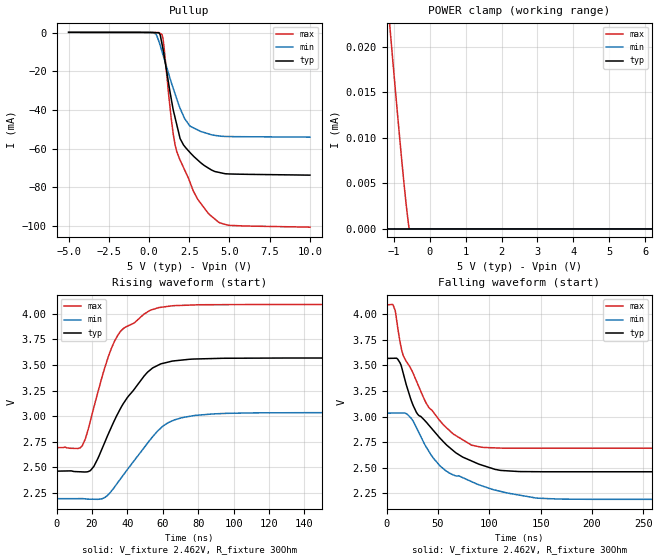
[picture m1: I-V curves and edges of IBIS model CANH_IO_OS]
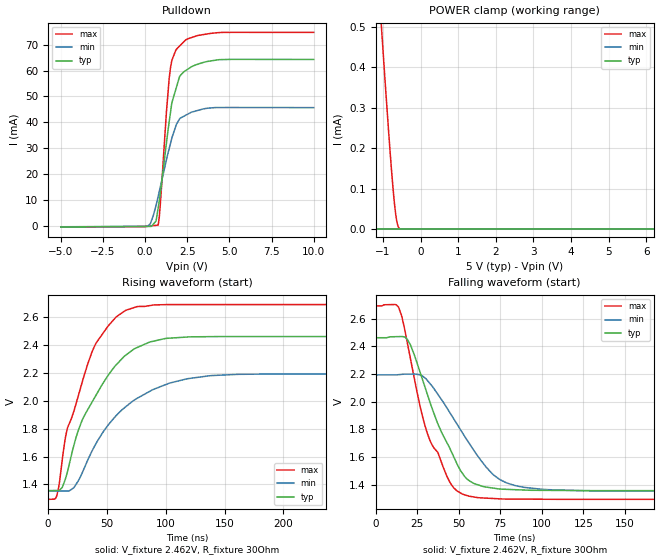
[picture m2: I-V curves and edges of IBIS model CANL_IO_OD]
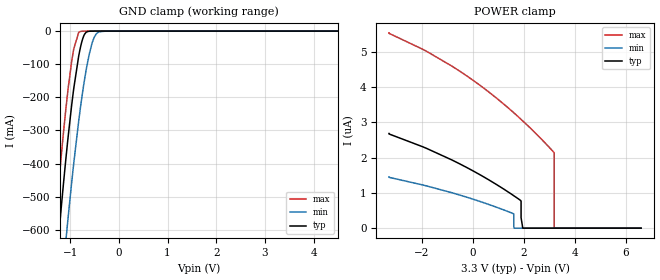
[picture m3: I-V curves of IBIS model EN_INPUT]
| Texas Instruments Incorporated
| TCAN1043Ax-Q1 Fault Protected CAN Transceiver with CAN FD
| Marketing part#   Digital Voltage Range   Package-type   #pins
| TCAN1043A-Q1   2.8V - 40V   SOIC , VSON   14
[IBIS Ver]   4.1
[File name]   tcan1043a-q1.ibs
[File Rev]   1.0
[Date]   12/13/2021
[Source]
| Texas Instruments Incorporated.
| Analog-eLab Design Center, HPA
| 12500 TI Blvd
| Dallas, TX -75243
[Notes]   Revision History:
| Rev 1.0: 12/13/2021
| - Initial version of the model
| - Model generated from simulations in SPECTRE
| - Model matched to SPICE simulation
| - C_comp although listed in numerical order of value are
|   obtained from varying PVT conditions. For PVT conditions for
|   each specific value refer the buffer description under
|   respective [Model]. IBIS model user is responsible for using
|   appropriate C_comp to simulate for Signal Integrity.
| - Notes regarding combined Non-monotonicity of various models
|   have been reviewed and considered minor and can be ignored.
| - For IBIS simulation of CANH-CANL differential pair, it is recommended
|   to use a capacitor(C) at common mode terminal with C >= 4.7nF
[Disclaimer]
| This model is designed as an aid for customers of Texas Instruments.
| TI and its licensors and suppliers make no warranties, either expressed
| or implied, with respect to this  model, including the warranties of
| merchantability or fitness for a particular purpose. The model is
| provided solely on an "as is" basis. The entire risk as to its quality
| and performance is with the customer.
[Copyright]
(C) Copyright 2017 Texas Instruments Incorporated.All rights reserved.
|   TCAN1043A-Q1_D
[Component]   TCAN1043A-Q1_D
[Manufacturer]   TI
[Package]   |14 SOIC
|   typ   min   max
R_pkg   0.2   0.16   0.24
L_pkg   1.5nH   1.2nH   1.8nH
C_pkg   0.4pF   0.32pF   0.48pF
[Pin]   signal_name   model_name   R_pin   L_pin   C_pin
1   TXD   TXD_INPUT   NA   NA   NA
2   GND   power   NA   NA   NA
3   VCC   power   NA   NA   NA
4   RXD   RXD_OUTPUT   NA   NA   NA
5   VIO   power   NA   NA   NA
6   EN   EN_INPUT   NA   NA   NA
7   INH   nc   NA   NA   NA
8   nFAULT   NFAULT_OUTPUT   NA   NA   NA
9   WAKE   WAKE_INPUT   NA   NA   NA
10   VSUP   power   NA   NA   NA
11   NC   nc   NA   NA   NA
12   CANL   CANL_IO_OD   NA   NA   NA
13   CANH   CANH_IO_OS   NA   NA   NA
14   nSTB   NSTB_INPUT   NA   NA   NA
|   TCAN1043A-Q1_DMT
[Component]   TCAN1043A-Q1_DMT
[Manufacturer]   TI
[Package]   |14 VSON
|   typ   min   max
R_pkg   0.2   0.16   0.24
L_pkg   1.5nH   1.2nH   1.8nH
C_pkg   0.4pF   0.32pF   0.48pF
[Pin]   signal_name   model_name   R_pin   L_pin   C_pin
1   TXD   TXD_INPUT   NA   NA   NA
2   GND   power   NA   NA   NA
3   VCC   power   NA   NA   NA
4   RXD   RXD_OUTPUT   NA   NA   NA
5   VIO   power   NA   NA   NA
6   EN   EN_INPUT   NA   NA   NA
7   INH   nc   NA   NA   NA
8   nFAULT   NFAULT_OUTPUT   NA   NA   NA
9   WAKE   WAKE_INPUT   NA   NA   NA
10   VSUP   power   NA   NA   NA
11   NC   nc   NA   NA   NA
12   CANL   CANL_IO_OD   NA   NA   NA
13   CANH   CANH_IO_OS   NA   NA   NA
14   nSTB   NSTB_INPUT   NA   NA   NA
|   TCAN1043A-Q1_DYY
[Component]   TCAN1043A-Q1_DYY
[Manufacturer]   TI
[Package]   |14 SOT
|   typ   min   max
R_pkg   0.2   0.16   0.24
L_pkg   1.5nH   1.2nH   1.8nH
C_pkg   0.4pF   0.32pF   0.48pF
[Pin]   signal_name   model_name   R_pin   L_pin   C_pin
1   TXD   TXD_INPUT   NA   NA   NA
2   GND   power   NA   NA   NA
3   VCC   power   NA   NA   NA
4   RXD   RXD_OUTPUT   NA   NA   NA
5   VIO   power   NA   NA   NA
6   EN   EN_INPUT   NA   NA   NA
7   INH   nc   NA   NA   NA
8   nFAULT   NFAULT_OUTPUT   NA   NA   NA
9   WAKE   WAKE_INPUT   NA   NA   NA
10   VSUP   power   NA   NA   NA
11   NC   nc   NA   NA   NA
12   CANL   CANL_IO_OD   NA   NA   NA
13   CANH   CANH_IO_OS   NA   NA   NA
14   nSTB   NSTB_INPUT   NA   NA   NA
| Models and submodels in the file (8): CANH_IO_OS (I/O_open_source), CANL_IO_OD (I/O_open_drain), EN_INPUT (Input), NFAULT_OUTPUT (3-state), NSTB_INPUT (Input), RXD_OUTPUT (3-state), TXD_INPUT (Input), WAKE_INPUT (Input)
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|   CANH_IO_OS Model
[Model]   CANH_IO_OS
Model_type   I/O_open_source
Polarity   Inverting
Enable   Active-High
Vinl = 0.5
Vinh = 0.9
Vmeas = 2.85
Vref = 2.462
Cref = 100pF
Rref = 30
|   typ   min   max
C_comp   11.441pF   10.949pF   11.932pF
|  Where Nom  PVT is Nominal Process,   5V,  27C
|   Fast PVT is Strong Process,   5.5V, -55C
|   Slow PVT is Weak Process,   4.5V, 150C
[Voltage Range]   5   4.5   5.5
|Junction Temperature
[Temperature Range]   27   150   -55
[Pullup Reference]   5   4.5   5.5
[Pulldown Reference]   0   0   0
[Power Clamp Reference]   5   4.5   5.5
[GND Clamp Reference]   0   0   0
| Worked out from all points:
|   slope of the pullup table from 0 to 0.75 V, typ, clamps not added: 207 ohm
|   falling waveform, V_fixture 2.462V, R_fixture 30Ohm: 20-80 % time 44.9ns typ, 53.4ns min, 39.2ns max; typ from 3.57 V to 2.46 V
|   rising waveform, V_fixture 2.462V, R_fixture 30Ohm: 20-80 % time 21.8ns typ, 22.8ns min, 16.1ns max; typ from 2.46 V to 3.57 V
[GND Clamp]
|   Voltage   I(typ)   I(min)   I(max)
-5V       0A         0A         0A
0V        0A         0A         0A
10V       0A         0A         0A
[Pullup]
|   Voltage   I(typ)   I(min)   I(max)
-5V       231.5uA    216.7uA    240.7uA
261.7mV   108uA      118.7uA    208.9uA
623.2mV   -9.522uA   -4.697mA   62.03uA
807.8mV   -5.906mA   -9.762mA   -930uA
934mV     -11.68mA   -13.29mA   -7.556mA
1.376V    -34.04mA   -25.58mA   -44.24mA
1.631V    -44.41mA   -31.97mA   -58.63mA
2.147V    -58.17mA   -43.24mA   -69.86mA
3.011V    -65.81mA   -50.27mA   -86.05mA
3.659V    -69.93mA   -52.25mA   -93.32mA
4.927V    -73.11mA   -53.73mA   -99.73mA
10V       -73.75mA   -54.05mA   -100.7mA
[POWER Clamp]
|   Voltage   I(typ)   I(min)   I(max)
-5V       147.1uA    97.29uA    209.7uA
-3.376V   78.29uA    39.94uA    130uA
-2.799V   54.44uA    20.87uA    102.2uA
-2.262V   32.83uA    4.577uA    76.39uA
-2.046V   24.12uA    0A         66.11uA
-2.01V    22.67uA    0A         64.41uA
-1.457V   2.561uA    0A         38.3uA
-1.36V    1.982nA    0A         33.72uA
-1.112V   0A         0A         22.14uA
-730.4mV  0A         0A         5.465uA
-573.8mV  0A         0A         0A
10V       0A         0A         0A
[Ramp]
R_load = 30
|   typ   min   max
dV/dt_r   0.663639/2.16889e-08   0.504683/2.27721e-08   0.839382/1.59848e-08
dV/dt_f   0.663639/4.47213e-08   0.504683/5.30098e-08   0.839383/3.92519e-08
[Falling Waveform]
V_fixture = 2.462V
V_fixture_min = 2.193V
V_fixture_max = 2.692V
R_fixture = 30Ohm
C_fixture = 0F
|   Time   V(typ)   V(min)   V(max)
0s        3.568V     3.034V     4.091V
8.333ns   3.57V      3.035V     4.032V
14.51ns   3.483V     3.035V     3.653V
19.95ns   3.282V     3.024V     3.526V
28.81ns   3.044V     2.895V     3.351V
40.81ns   2.92V      2.666V     3.092V
60.08ns   2.708V     2.456V     2.874V
92.08ns   2.529V     2.327V     2.702V
168ns     2.462V     2.195V     2.692V
1us       2.462V     2.193V     2.692V
[Rising Waveform]
V_fixture = 2.462V
V_fixture_min = 2.193V
V_fixture_max = 2.692V
R_fixture = 30Ohm
C_fixture = 0F
|   Time   V(typ)   V(min)   V(max)
0s        2.462V     2.193V     2.692V
14.51ns   2.455V     2.194V     2.709V
17.46ns   2.456V     2.189V     2.845V
21.07ns   2.508V     2.187V     3.085V
29.43ns   2.832V     2.237V     3.59V
36.05ns   3.072V     2.385V     3.826V
51.41ns   3.43V      2.736V     4.019V
65.54ns   3.538V     2.955V     4.079V
112.6ns   3.567V     3.032V     4.091V
1us       3.568V     3.034V     4.091V
|   CANL_IO_OD Model
[Model]   CANL_IO_OD
Model_type   I/O_open_drain
Polarity   Non-Inverting
Enable   Active-High
Vinl = 0.5
Vinh = 0.9
Vmeas = 1.8
Vref = 2.462
Cref = 100pF
Rref = 30
|   typ   min   max
C_comp   11.441pF   10.949pF   11.932pF
|  Where Nom  PVT is Nominal Process,   5V,  27C
|   Fast PVT is Strong Process,   5.5V, -55C
|   Slow PVT is Weak Process,   4.5V, 150C
[Voltage Range]   5   4.5   5.5
|Junction Temperature
[Temperature Range]   27   150   -55
[Pullup Reference]   5   4.5   5.5
[Pulldown Reference]   -0   0   -0
[Power Clamp Reference]   5   4.5   5.5
[GND Clamp Reference]   0   0   0
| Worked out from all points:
|   slope of the pulldown table from 0 to 0.75 V, typ, clamps not added: 122 ohm
|   POWER clamp passes 1 mA (typ) near -2.33 V on its own axis
|   falling waveform, V_fixture 2.462V, R_fixture 30Ohm: 20-80 % time 21.9ns typ, 27.9ns min, 20ns max; typ from 2.46 V to 1.36 V
|   rising waveform, V_fixture 2.462V, R_fixture 30Ohm: 20-80 % time 37.2ns typ, 46.1ns min, 28.6ns max; typ from 1.36 V to 2.46 V
[Pulldown]
|   Voltage   I(typ)   I(min)   I(max)
-5V       -375.4uA   -308.4uA   -451.2uA
131mV     -170uA     -116.4uA   -123.6uA
651.1mV   1.944mA    7.976mA    264.7uA
776.6mV   7.041mA    11.48mA    358.4uA
904.4mV   12.67mA    15.15mA    8.49mA
1.265V    31.94mA    25.51mA    43.97mA
1.508V    43.91mA    31.89mA    61.21mA
1.817V    52.64mA    38.46mA    67.79mA
2.051V    57.82mA    41.39mA    69.49mA
2.406V    59.99mA    42.76mA    71.83mA
4.38V     64.21mA    45.72mA    74.67mA
10V       64.3mA     45.71mA    74.75mA
[GND Clamp]
|   Voltage   I(typ)   I(min)   I(max)
-5V       0A         0A         0A
0V        0A         0A         0A
10V       0A         0A         0A
[POWER Clamp]
|   Voltage   I(typ)   I(min)   I(max)
-5V       4.492mA    2.914mA    6.422mA
-2.941V   1.781mA    653.9uA    3.311mA
-2.703V   1.476mA    407.7uA    2.953mA
-2.4V     1.086mA    132.9uA    2.498mA
-2.124V   738.5uA    5.645uA    2.085mA
-1.895V   454.5uA    4.17uA     1.743mA
-1.462V   25.53uA    1.377uA    1.104mA
-1.249V   0A         4.387nA    791.4uA
-1.017V   0A         0A         462.9uA
-710.9mV  0A         0A         75.75uA
-553.4mV  0A         0A         0A
10V       0A         0A         0A
[Ramp]
R_load = 30
|   typ   min   max
dV/dt_r   0.663744/3.72064e-08   0.504631/4.59502e-08   0.83937/2.86431e-08
dV/dt_f   0.663744/2.18742e-08   0.504631/2.78671e-08   0.83937/1.99272e-08
[Falling Waveform]
V_fixture = 2.462V
V_fixture_min = 2.193V
V_fixture_max = 2.692V
R_fixture = 30Ohm
C_fixture = 0F
|   Time   V(typ)   V(min)   V(max)
0s        2.462V     2.193V     2.692V
13.84ns   2.47V      2.195V     2.683V
19.07ns   2.451V     2.199V     2.428V
26.93ns   2.207V     2.192V     1.959V
33.13ns   1.981V     2.125V     1.708V
46.84ns   1.606V     1.879V     1.379V
61.59ns   1.398V     1.605V     1.305V
78.87ns   1.365V     1.412V     1.295V
125.2ns   1.356V     1.355V     1.293V
1us       1.356V     1.352V     1.293V
[Rising Waveform]
V_fixture = 2.462V
V_fixture_min = 2.193V
V_fixture_max = 2.692V
R_fixture = 30Ohm
C_fixture = 0F
|   Time   V(typ)   V(min)   V(max)
0s        1.356V     1.352V     1.293V
7.199ns   1.357V     1.352V     1.315V
11.9ns    1.377V     1.353V     1.57V
16.18ns   1.484V     1.353V     1.798V
25.7ns    1.79V      1.427V     2.038V
39.09ns   2.017V     1.669V     2.387V
57.53ns   2.256V     1.892V     2.6V
75.33ns   2.382V     2.017V     2.676V
161.6ns   2.462V     2.191V     2.692V
1us       2.462V     2.193V     2.692V
|   EN_INPUT Model
[Model]   EN_INPUT
Model_type   Input
Vinl = 0.99
Vinh = 2.31
|   typ   min   max
C_comp   1.526pF   1.317pF   1.651pF
|  Where Nom  PVT is Nominal Process,   3.3V,  27C
|   Fast PVT is Strong Process,   5.5V, -55C
|   Slow PVT is Weak Process,   2.8V, 150C
[Model spec]
|subparameter
Vinl   0.990   0.840   1.650
Vinh   2.310   1.960   3.850
[Voltage Range]   3.3   2.8   5.5
|Junction Temperature
[Temperature Range]   27   150   -55
[Power Clamp Reference]   3.3   2.8   5.5
[GND Clamp Reference]   0   0   0
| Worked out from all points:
|   GND clamp passes 1 mA (typ) near -0.63 V on its own axis
[GND Clamp]
|   Voltage   I(typ)   I(min)   I(max)
-3.3V     -4.563A    -4.77A     -4.442A
-1.327V   -775mA     -1.025A    -620.1mA
-1.248V   -639mA     -890mA     -482.8mA
-1.182V   -530mA     -780.6mA   -374.1mA
-1.087V   -383.2mA   -630.1mA   -232.3mA
-1.045V   -322.7mA   -566.2mA   -176.6mA
-927.2mV  -173.8mA   -399.8mA   -54.18mA
-797.6mV  -54.91mA   -240.4mA   -1.604mA
-710.6mV  -11.23mA   -151.5mA   -191.2uA
-602.7mV  -443.2uA   -66.49mA   -16.11uA
-408.6mV  -2.826uA   -2.179mA   -519.7nA
6.6V      0A         0A         0A
[POWER Clamp]
|   Voltage   I(typ)   I(min)   I(max)
-3.3V     2.684uA    1.455uA    5.537uA
1.443V    996.2nA    451.6nA    3.372uA
1.862V    789.6nA    0A         3.101uA
1.887V    771.1nA    0A         3.084uA
1.887V    743.9nA    0A         3.084uA
1.887V    298.2nA    0A         3.084uA
1.954V    0A         0A         3.039uA
3.184V    0A         0A         2.142uA
3.188V    0A         0A         2.116uA
3.188V    0A         0A         1.856uA
3.188V    0A         0A         0A
6.6V      0A         0A         0A
